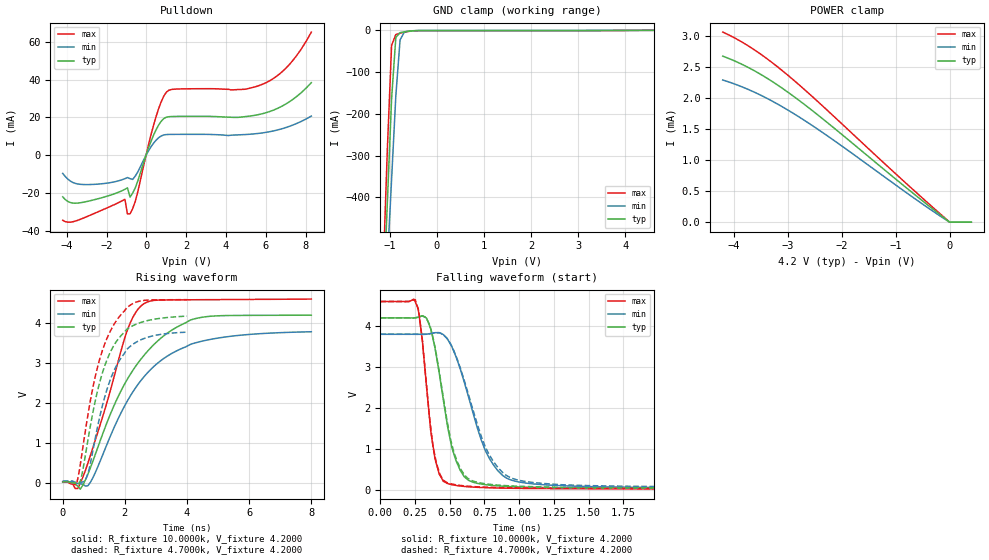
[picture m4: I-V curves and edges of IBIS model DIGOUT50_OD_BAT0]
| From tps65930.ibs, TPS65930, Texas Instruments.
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|   Model DIGOUT50_OD_BAT0
[Model]   DIGOUT50_OD_BAT0
Model_type   3-state
Polarity   Non-Inverting
Enable   Active-Low
Vmeas =   2.1000V
Cref =  30.0000pF
Rref = 100.0000M
Vref =  0.000V
C_comp   0.4246pF   0.4608pF   0.4132pF
[Temperature Range]   25.0000   0.1250k   -40.0000
[Pullup Reference]   4.2000V   3.8000V   4.6000V
[Pulldown Reference]   0.000V   0.000V   0.000V
[POWER Clamp Reference]   4.2000V   3.8000V   4.6000V
[GND Clamp Reference]   0.000V   0.000V   0.000V
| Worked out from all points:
|   slope of the pulldown table from 0 to 0.63 V, typ, clamps not added: 40.4 ohm
|   GND clamp passes 1 mA (typ) near -0.48 V on its own axis
|   POWER clamp passes 1 mA (typ) near -1.42 V on its own axis
|   rising waveform, R_fixture 10.0000k, V_fixture 4.2000: 20-80 % time 1.69ns typ, 1.78ns min, 1.03ns max; typ from 0.013 V to 4.18 V
|   falling waveform, R_fixture 10.0000k, V_fixture 4.2000: 20-80 % time 132ps typ, 215ps min, 84.6ps max; typ from 4.2 V to 0.025 V
|   rising waveform, R_fixture 4.7000k, V_fixture 4.2000: 20-80 % time 814ps typ, 830ps min, 799ps max; typ from 0.029 V to 4.16 V
|   falling waveform, R_fixture 4.7000k, V_fixture 4.2000: 20-80 % time 134ps typ, 224ps min, 85ps max; typ from 4.2 V to 0.043 V
[Pulldown]
| voltage   I(typ)   I(min)   I(max)
-4.2V     -21.97mA   -9.563mA   -34.32mA
-3.29V    -25.03mA   -15.36mA   -33.72mA
-1.08V    -17.98mA   -12.36mA   -23.22mA
-950mV    -17.21mA   -11.76mA   -30.99mA
-820mV    -22.04mA   -12.33mA   -30.93mA
-560mV    -17.27mA   -11.04mA   -24.49mA
480mV     13.34mA    7.894mA    20.21mA
870mV     19.36mA    10.74mA    31.19mA
1.13V     20.37mA    11.01mA    34.37mA
5.81V     21.93mA    11.81mA    37.44mA
7.11V     27.8mA     15.03mA    47.18mA
8.28V     38.35mA    20.72mA    65.08mA
[Pullup]
| voltage   I(typ)   I(min)   I(max)
-4.08V    0A         0A         0A
-3.95V    0A         0A         0A
-3.82V    0A         0A         0A
8.27V     0A         0A         0A
[GND_clamp]
| voltage   I(typ)   I(min)   I(max)
-4.2V     -9.128A    -7.565A    -10.64A
-1.14V    -661.4mA   -757.1mA   -581.1mA
-1.05V    -412.4mA   -556.9mA   -285.5mA
-960mV    -163.5mA   -356.7mA   -35.94mA
-870mV    -16.94mA   -156.5mA   -9.991mA
-780mV    -5.49mA    -22.82mA   -6.947mA
-690mV    -3.486mA   -4.275mA   -4.545mA
-600mV    -2.115mA   -1.869mA   -2.613mA
-330mV    -616uA     -378.4uA   -823.8uA
4.6V      0A         0A         0A
[POWER_clamp]
| voltage   I(typ)   I(min)   I(max)
-4.2V     2.674mA    2.29mA     3.062mA
-3.9V     2.566mA    2.2mA      2.93mA
-3.6V     2.432mA    2.088mA    2.768mA
-3.25V    2.247mA    1.934mA    2.547mA
-2.9V     2.034mA    1.756mA    2.297mA
-2.25V    1.594mA    1.383mA    1.79mA
-650mV    446.7uA    382uA      502.6uA
0V        89.58pA    3.972nA    77.61pA
400mV     0A         0A         0A
[Ramp]
| variable   typ   min   max
dV/dt_r   42.8884u/13.5627p  0.2673m/0.3000n   2.3015u/0.1114n
dV/dt_f   0.5742/0.2193n   0.2788/0.2678n   0.9927/0.1664n
R_load = 50.0000
[Rising Waveform]
R_fixture = 10.0000k
V_fixture = 4.2000
V_fixture_min = 3.8000
V_fixture_max = 4.6000
| time   V(typ)   V(min)   V(max)
0s        13.44mV    19.47mV    10.09mV
404ps     -39.5mV    -14.1mV    -149.3mV
565.7ps   -165.1mV   -29.71mV   -15.7mV
888.9ps   363.7mV    2.952mV    672.5mV
2.02ns    2.503V     1.957V     3.676V
2.263ns   2.812V     2.274V     4.139V
2.586ns   3.153V     2.618V     4.458V
3.313ns   3.706V     3.135V     4.566V
4.283ns   4.102V     3.496V     4.571V
8ns       4.185V     3.771V     4.588V
[Falling Waveform]
R_fixture = 10.0000k
V_fixture = 4.2000
V_fixture_min = 3.8000
V_fixture_max = 4.6000
| time   V(typ)   V(min)   V(max)
0s        4.2V       3.8V       4.6V
272.7ps   4.218V     3.8V       4.439V
333.3ps   4.194V     3.801V     2.514V
393.9ps   3.473V     3.839V     759.9mV
484.8ps   1.543V     3.681V     149.6mV
545.5ps   708.8mV    3.254V     104.7mV
606.1ps   312.3mV    2.616V     79.88mV
757.6ps   123.3mV    951.1mV    50.48mV
939.4ps   76.13mV    239.8mV    35.95mV
3ns       25.22mV    42.05mV    13.44mV
[Rising Waveform]
R_fixture = 4.7000k
V_fixture = 4.2000
V_fixture_min = 3.8000
V_fixture_max = 4.6000
| time   V(typ)   V(min)   V(max)
0s        28.61mV    41.52mV    21.46mV
444.4ps   -20.23mV   5.192mV    -31.5mV
565.7ps   36.13mV    6.619mV    450.5mV
767.7ps   860mV      130.7mV    1.484V
969.7ps   1.746V     793.2mV    2.37V
1.212ns   2.567V     1.713V     3.142V
1.455ns   3.126V     2.401V     3.658V
1.737ns   3.538V     2.933V     4.059V
2.465ns   3.99V      3.551V     4.535V
4ns       4.162V     3.761V     4.574V
[Falling Waveform]
R_fixture = 4.7000k
V_fixture = 4.2000
V_fixture_min = 3.8000
V_fixture_max = 4.6000
| time   V(typ)   V(min)   V(max)
0s        4.2V       3.8V       4.6V
252.5ps   4.2V       3.8V       4.644V
303ps     4.252V     3.798V     3.659V
378.8ps   3.738V     3.829V     1.08V
479.8ps   1.707V     3.705V     177mV
530.3ps   909.8mV    3.395V     129.3mV
606.1ps   359.2mV    2.658V     93.51mV
757.6ps   145.2mV    1.039V     62.58mV
934.3ps   94.65mV    299.9mV    47.93mV
2.5ns     43.39mV    69.26mV    27.14mV
